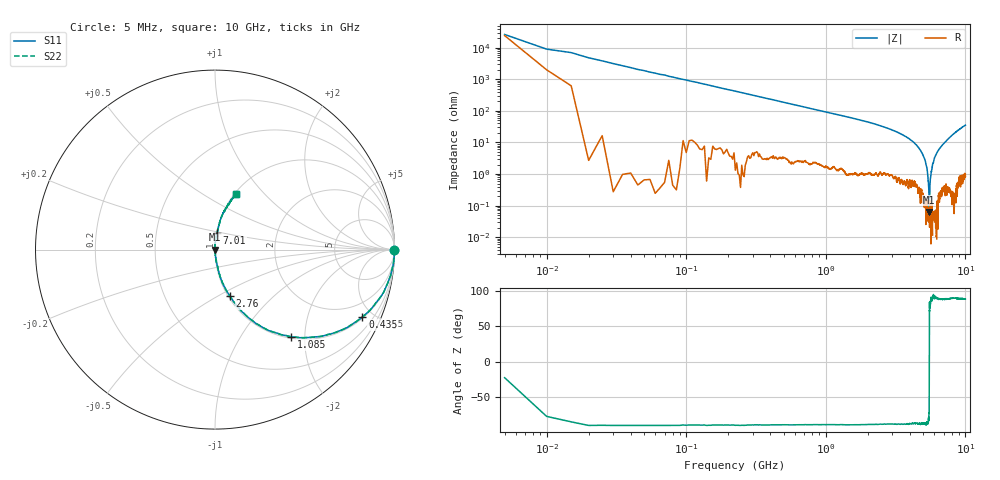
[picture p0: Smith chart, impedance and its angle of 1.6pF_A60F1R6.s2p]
! Amotech Co.,Ltd.
! http://www.amotech.co.kr/
! Part Number: A60F1R6
! These Parameters are Measured in Series Mode Connection
! Operation Temp=25[degC], DC Bias Voltage=0[V]
! Freq. Start=5[MHz] Stop=10[GHz], 2000[Steps]
! Date: Monday, July 20, 2020, 03:17:09
# GHZ S RI R 50.000000
!Freq.(Hz) S11(Real) S11(Imag) S21(Real) S21(Imag) S12(Real) S12(Imag) S22(Real) S22(Imag)
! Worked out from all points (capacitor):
!   2000 points, 5 MHz to 10 GHz, reference 50 ohm
!   read as one part in series: C = 1.68 pF near 55 MHz
!   lowest |Z| = 62.6 mohm at 5.515 GHz (marker M1)
!   series resonance near 5.515 GHz, so ESL is about 490 pH
!   S11 on the Smith chart (normalised r, x): 5 MHz: open; 435 MHz: 1.07, -4.35; 1.085 GHz: 1.03, -1.71; 2.76 GHz: 1.02, -0.57; 7.01 GHz: 1.01, +0.19; 10 GHz: 1.02, +0.71
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0.005  0.9965 -0.00144  0.00347 0.00144  0.00347 0.00144  0.9965 -0.00144
0.065  0.9952 -0.0691  0.00481 0.0691  0.00481 0.0691  0.9952 -0.0691
0.125  0.982 -0.1288  0.018 0.1288  0.018 0.1288  0.982 -0.1288
0.245  0.9375 -0.2416  0.0625 0.2416  0.0625 0.2416  0.9375 -0.2416
0.435  0.8216 -0.375  0.1784 0.375  0.1784 0.375  0.8216 -0.375
1.085  0.4228 -0.4858  0.5772 0.4858  0.5772 0.4858  0.4228 -0.4858
1.675  0.2332 -0.4143  0.7668 0.4143  0.7668 0.4143  0.2332 -0.4143
2.76  0.0832 -0.2592  0.9168 0.2592  0.9168 0.2592  0.0832 -0.2592
3.34  0.0451 -0.189  0.9549 0.189  0.9549 0.189  0.0451 -0.189
4.45  0.0114 -0.0834  0.9886 0.0834  0.9886 0.0834  0.0114 -0.0834
5.005  0.00348 -0.0366  0.9965 0.0366  0.9965 0.0366  0.00348 -0.0366
5.31  0.00137 -0.0144  0.9986 0.0144  0.9986 0.0144  0.00137 -0.0144
5.415  0.000563 -0.0059  0.9994 0.0059  0.9994 0.0059  0.000563 -0.0059
5.48  0.000781 -0.0026  0.9992 0.0026  0.9992 0.0026  0.000781 -0.0026
5.515  0.000622 -7.1e-05  0.9994 7.1e-05  0.9994 7.1e-05  0.000622 -7.1e-05
5.645  0.000467 0.00883  0.9995 -0.00883  0.9995 -0.00883  0.000467 0.00883
5.825  0.000235 0.0208  0.9998 -0.0208  0.9998 -0.0208  0.000235 0.0208
6.2  0.00167 0.0447  0.9983 -0.0447  0.9983 -0.0447  0.00167 0.0447
6.67  0.00797 0.0722  0.992 -0.0722  0.992 -0.0722  0.00797 0.0722
7.01  0.0113 0.0917  0.9887 -0.0917  0.9887 -0.0917  0.0113 0.0917
8.335  0.0391 0.1902  0.9609 -0.1902  0.9609 -0.1902  0.0391 0.1902
10  0.1183 0.3094  0.8817 -0.3094  0.8817 -0.3094  0.1183 0.3094
